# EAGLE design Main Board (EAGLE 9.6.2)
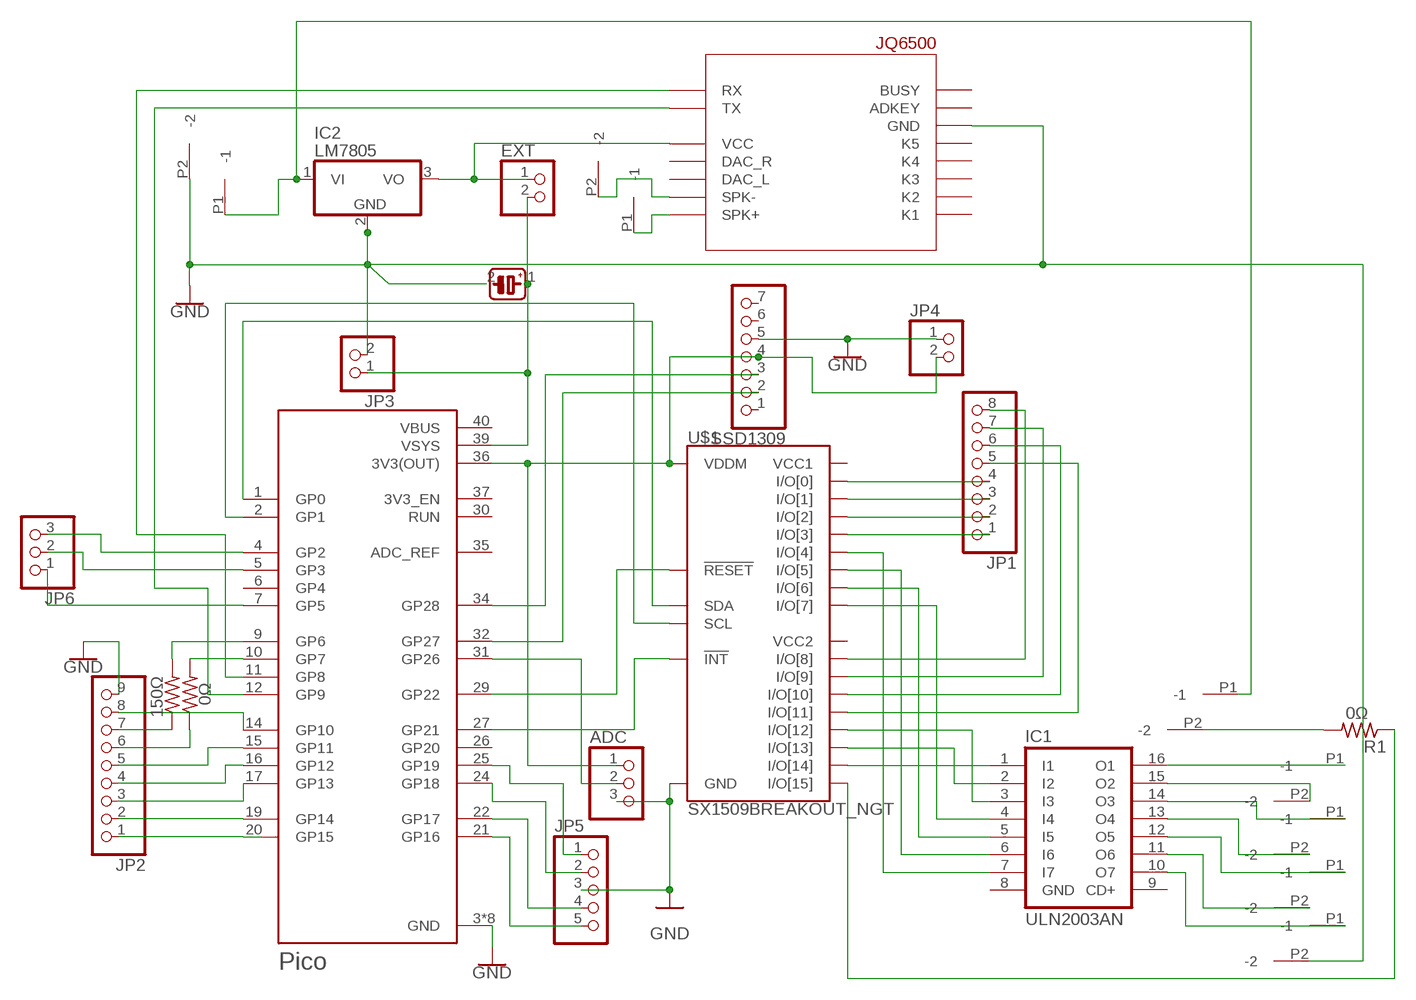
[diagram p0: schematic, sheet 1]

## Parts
ADC  PINHD-1X3  [1X03]
EXT  PINHD-1X2  [1X02]
IC1  ULN2003AN  [DIL16]
IC2  LM7805  7805TV  [TO220V]
JP1  PINHD-1X8  [1X08]
JP2  PINHD-1X9  [1X09]
JP3  PINHD-1X2  [1X02]
JP4  PINHD-1X2  [1X02]
JP5  PINHD-1X5  [1X05]
JP6  PINHD-1X3  [1X03]
R1  0Ω  R-US_0207/15  [0207/15]
R3  150Ω  R-US_0207/12  [0207/12]
R4  0Ω  R-US_0207/12  [0207/12]
SSD1309  PINHD-1X7  [1X07]
U1  Pico  RASPBERRY_PICOTH  [PICO-PKG-TH]
U$1  SX1509BREAKOUT_NGT  [BREAKOUT_NGT]
U$2  JQ6500  [JQ6500]
U$3  CONNECTORSCREWLESS2POS  [CONNECTORSCREWLESS2POS]
U$4  CONNECTORSCREWLESS2POS  [CONNECTORSCREWLESS2POS]
U$5  CONNECTORSCREWLESS2POS  [CONNECTORSCREWLESS2POS]
U$6  CONNECTORSCREWLESS2POS  [CONNECTORSCREWLESS2POS]
U$7  CONNECTORSCREWLESS2POS  [CONNECTORSCREWLESS2POS]
U$8  CONNECTORSCREWLESS2POS  [CONNECTORSCREWLESS2POS]
U$9  CONNECTORSCREWLESS2POS  [CONNECTORSCREWLESS2POS]
U$10  CAPACITOR_TANTALUM_RADIAL_10UF  [CAPACITOR_TANTALUM_RADIAL_10UF]

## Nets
GND: ADC.3 IC2.2(GND) JP2.9 JP3.2 JP4.1 JP5.3 SSD1309.5 U1.3(GND) U1.8(GND) U1.13(GND) U1.18(GND) U1.23(GND) U1.28(GND) U1.33(GND) U1.38(GND) U$1.GND U$1.GND3(GND) U$1.GND4(GND) U$2.GND1(GND) U$2.GND2(GND) U$3.P2(-2) U$8.P2(-2) U$10.2
N$1: JP1.4 U$1.I/O[0]
N$2: JP1.3 U$1.I/O[1]
N$3: JP1.1 U$1.I/O[3]
N$4: JP1.2 U$1.I/O[2]
N$5: JP1.8 U$1.I/O[8]
N$6: JP1.5 U$1.I/O[11]
N$7: JP1.7 U$1.I/O[9]
N$8: JP1.6 U$1.I/O[10]
N$9: IC1.3(I3) U$1.I/O[12]
N$10: IC1.2(I2) U$1.I/O[13]
N$11: IC1.1(I1) U$1.I/O[14]
N$12: IC1.4(I4) U$1.I/O[7]
N$13: IC1.5(I5) U$1.I/O[6]
N$14: IC1.6(I6) U$1.I/O[5]
N$15: IC1.7(I7) U$1.I/O[4]
N$16: IC2.1(VI) U$7.P1(-1) U$8.P1(-1)
N$17: R1.2 U$7.P2(-2)
N$18: EXT.1 IC2.3(VO) U$2.VCC
N$19: R4.2 U1.10(GP7)
N$20: SSD1309.3 U1.34(GP28)
N$21: R1.1 U$1.I/O[15]
N$22: IC1.16(O1) U$6.P1(-1)
N$23: IC1.15(O2) U$6.P2(-2)
N$24: IC1.14(O3) U$5.P1(-1)
N$25: IC1.13(O4) U$5.P2(-2)
N$26: IC1.12(O5) U$4.P1(-1)
N$27: IC1.11(O6) U$4.P2(-2)
N$28: IC1.10(O7) U$3.P1(-1)
N$29: ADC.1 JP4.2 SSD1309.4 U1.36(3V3(OUT)) U$1.VDDM
N$30: U1.1(GP0) U$1.SDA
N$31: U1.2(GP1) U$1.SCL
N$32: SSD1309.2 U1.32(GP27)
N$33: ADC.2 U1.31(GP26)
N$34: U1.29(GP22) U$1.!RESET
N$35: U1.27(GP21) U$1.!INT
N$36: U1.11(GP8) U$2.RX
N$37: U1.12(GP9) U$2.TX
N$38: U$2.SPK+ U$9.P1(-1)
N$39: U$2.SPK- U$9.P2(-2)
N$40: JP2.1 U1.20(GP15)
N$41: JP2.2 U1.19(GP14)
N$42: JP2.3 U1.17(GP13)
N$43: JP2.4 U1.16(GP12)
N$44: JP2.5 U1.15(GP11)
N$45: JP2.6 R4.1
N$46: R3.2 U1.9(GP6)
N$47: JP6.3 U1.4(GP2)
N$48: EXT.2 JP3.1 U1.39(VSYS) U$10.1
N$49: JP2.7 R3.1
N$50: JP6.2 U1.5(GP3)
N$51: JP2.8 U1.14(GP10)
N$52: JP5.1 U1.25(GP19)
N$53: JP5.2 U1.24(GP18)
N$54: JP5.4 U1.22(GP17)
N$55: JP5.5 U1.21(GP16)
N$56: JP6.1 U1.7(GP5)
Unconnected: IC1.9(CD+) SSD1309.1 SSD1309.6 SSD1309.7 U1.6(GP4) U1.26(GP20) U1.30(RUN) U1.35(ADC_REF) U1.37(3V3_EN) U$1.VCC1 U$1.VCC2 U$2.ADKEY U$2.BUSY U$2.DAC-L(DAC_L) U$2.DAC-R(DAC_R) U$2.K1 U$2.K2 U$2.K3 U$2.K4 U$2.K5

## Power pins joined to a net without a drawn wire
GND: IC1.8(GND)
VBUS: U1.40(VBUS)

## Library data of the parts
ADC JP6 = pinhead:PINHD-1X3: PIN HEADER
EXT JP3 JP4 = pinhead:PINHD-1X2: PIN HEADER
IC1 = uln-udn:ULN2003A: DRIVER ARRAY
IC2 = linear:78*: Positive VOLTAGE REGULATOR Source: http://cache.national.com/ds/LM/LM78L05.pdf http://www.fairchildsemi.com/ds/LM/LM7805.pdf
JP1 = pinhead:PINHD-1X8: PIN HEADER
JP2 = pinhead:PINHD-1X9: PIN HEADER
JP5 = pinhead:PINHD-1X5: PIN HEADER
R1 R3 R4 = rcl:R-US_: RESISTOR, American symbol; SPICEPREFIX: R
SSD1309 = pinhead:PINHD-1X7: PIN HEADER
U1 = RpiPico:RASPBERRY_PICO: Raspberry Pi Pico
U$1 = SX1509 Breakout:SX1509BREAKOUT_NGT
U$2 = JQ6500:JQ6500: JQ6500 MP3 Module
U$3-U$9 = Williams:CONNECTORSCREWLESS2POS
U$10 = Williams:CAPACITOR_TANTALUM_RADIAL_10UF

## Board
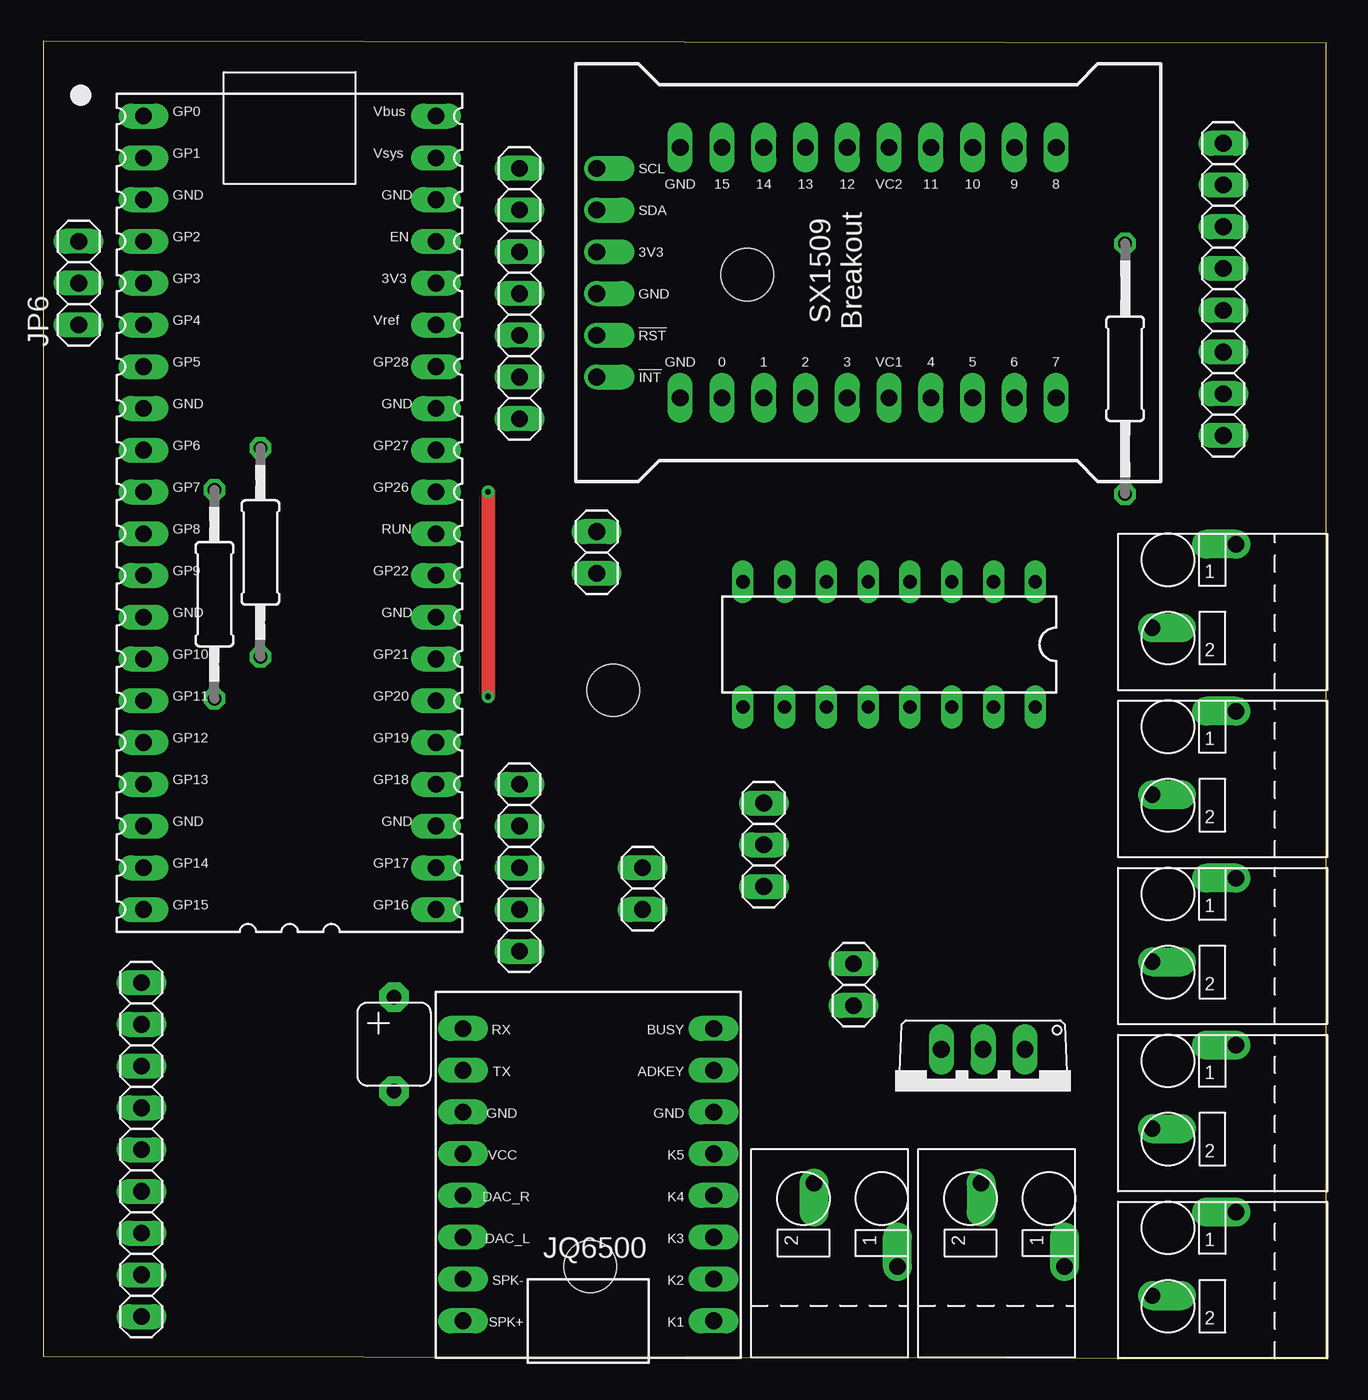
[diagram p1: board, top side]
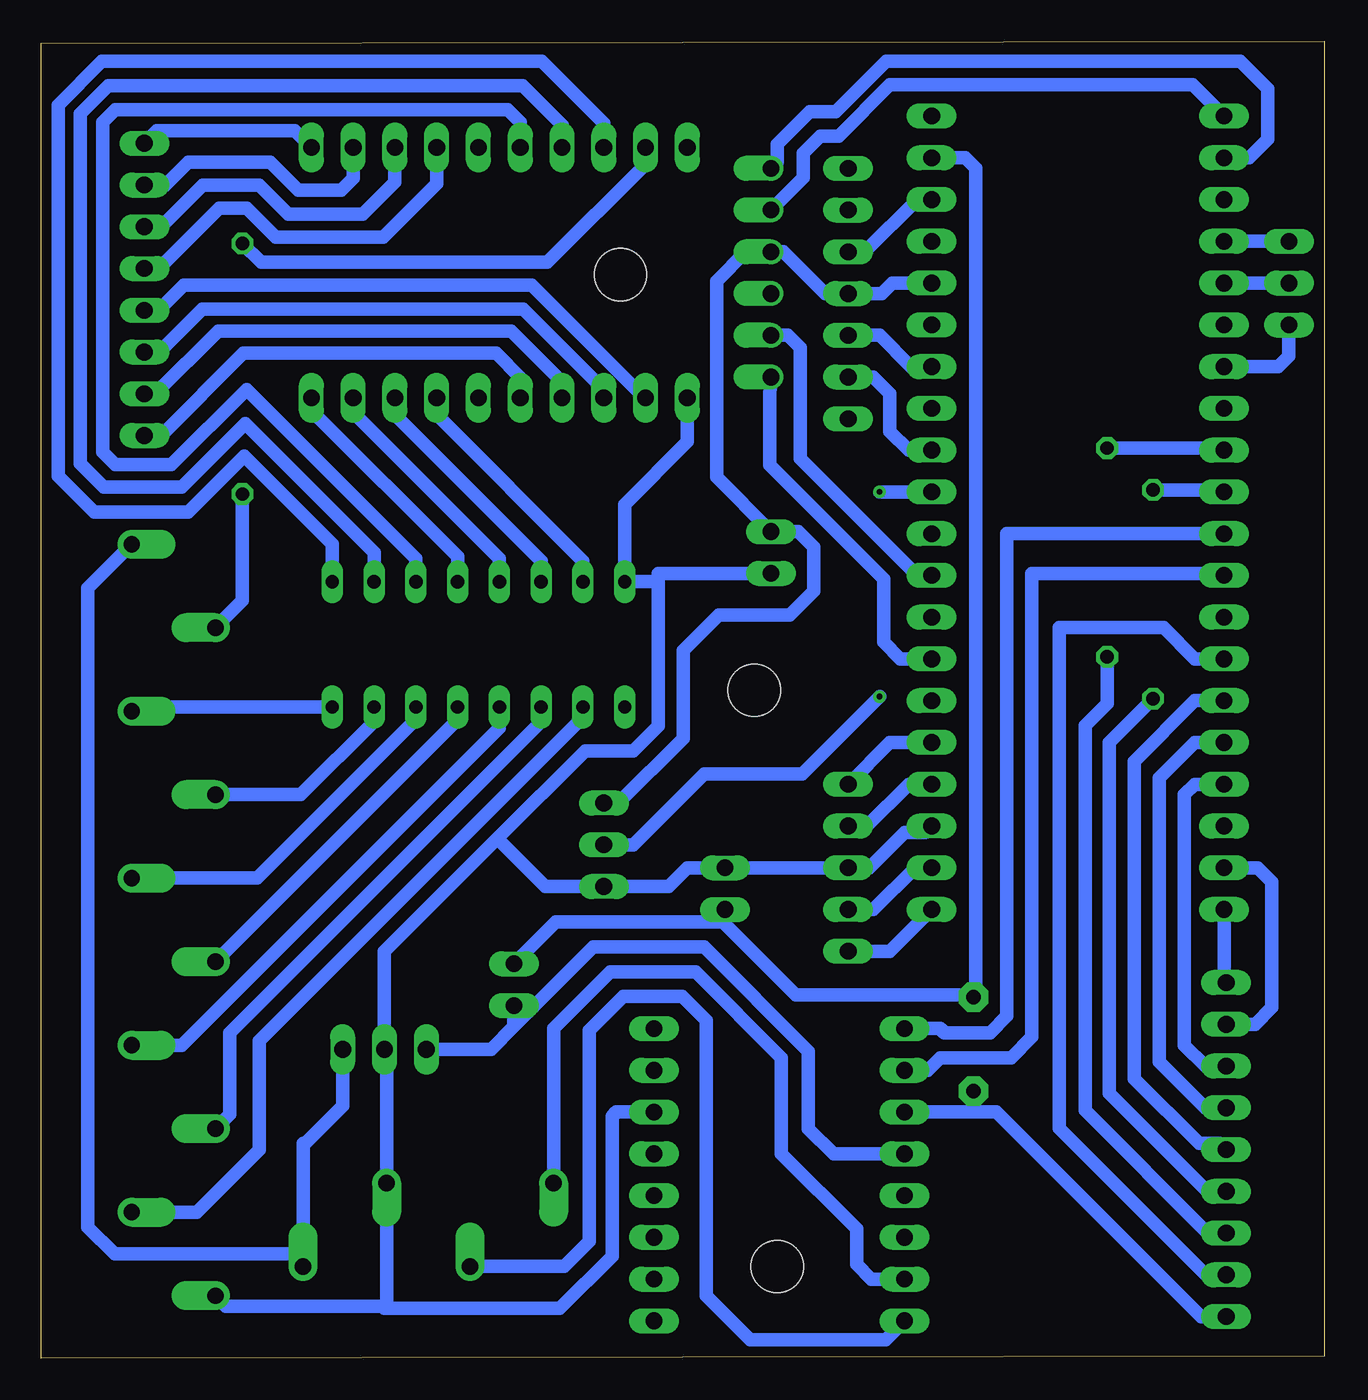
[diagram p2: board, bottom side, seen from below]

Size 78.03 x 80.13 mm. Coordinates in mm from the lower left corner, seen from the top.
Outline: 0,0.13 78.03,0 78.03,80 0,80.13 0,0.13
Copper layers (1*16): Top 0.035mm / dielectric 1.5mm / Bottom 0.035mm
Design rules "default *": minimum track width 6mil, minimum drill 0.35mm, track to track 6mil, track to pad 6mil, pad to pad 6mil, via to via 6mil, smd to smd 6mil, copper to edge 25mil, drill to drill 6mil, minimum pad ring 10mil, minimum via ring 8mil, stop-mask expansion 4mil, vias tented up to drill 0mil, thermal gap 10mil
Holes 3.17 mm at 34.67,40.64 42.8,65.91 33.27,5.59
tRestrict: area 29.9,35.9 to 39.4,45.4; area 38,61.2 to 47.6,70.7; area 28.5,0.8 to 38,10.4

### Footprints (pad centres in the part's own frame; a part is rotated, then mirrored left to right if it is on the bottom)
1X03 = drill 1.016 long: 1 -2.54,0; 2 0,0; 3 2.54,0
1X02 = drill 1.016 long: 1 -1.27,0; 2 1.27,0
DIL16 = drill 0.813 long: 1 -8.89,-3.81; 2 -6.35,-3.81; 3 -3.81,-3.81; 4 -1.27,-3.81; 5 1.27,-3.81; 6 3.81,-3.81; 7 6.35,-3.81; 8 8.89,-3.81; 9 8.89,3.81; 10 6.35,3.81; 11 3.81,3.81; 12 1.27,3.81; 13 -1.27,3.81; 14 -3.81,3.81; 15 -6.35,3.81; 16 -8.89,3.81
TO220V = drill 1.016 long: 1 -2.54,-2.54; 2 0,-2.54; 3 2.54,-2.54
1X08 = drill 1.016 long: 1 -8.89,0; 2 -6.35,0; 3 -3.81,0; 4 -1.27,0; 5 1.27,0; 6 3.81,0; 7 6.35,0; 8 8.89,0
1X09 = drill 1.016 long: 1 -10.16,0; 2 -7.62,0; 3 -5.08,0; 4 -2.54,0; 5 0,0; 6 2.54,0; 7 5.08,0; 8 7.62,0; 9 10.16,0
1X05 = drill 1.016 long: 1 -5.08,0; 2 -2.54,0; 3 0,0; 4 2.54,0; 5 5.08,0
0207/15 = drill 0.813 octagon: 1 -7.62,0; 2 7.62,0
0207/12 = drill 0.813 octagon: 1 -6.35,0; 2 6.35,0
1X07 = drill 1.016 long: 1 -7.62,0; 2 -5.08,0; 3 -2.54,0; 4 0,0; 5 2.54,0; 6 5.08,0; 7 7.62,0
PICO-PKG-TH = drill 1.016 long: 1 -8.89,24.13; 2 -8.89,21.59; 3 -8.89,19.05; 4 -8.89,16.51; 5 -8.89,13.97; 6 -8.89,11.43; 7 -8.89,8.89; 8 -8.89,6.35; 9 -8.89,3.81; 10 -8.89,1.27; 11 -8.89,-1.27; 12 -8.89,-3.81; 13 -8.89,-6.35; 14 -8.89,-8.89; 15 -8.89,-11.43; 16 -8.89,-13.97; 17 -8.89,-16.51; 18 -8.89,-19.05; 19 -8.89,-21.59; 20 -8.89,-24.13; 21 8.89,-24.13; 22 8.89,-21.59; 23 8.89,-19.05; 24 8.89,-16.51; 25 8.89,-13.97; 26 8.89,-11.43; 27 8.89,-8.89; 28 8.89,-6.35; 29 8.89,-3.81; 30 8.89,-1.27; 31 8.89,1.27; 32 8.89,3.81; 33 8.89,6.35; 34 8.89,8.89; 35 8.89,11.43; 36 8.89,13.97; 37 8.89,16.51; 38 8.89,19.05; 39 8.89,21.59; 40 8.89,24.13
BREAKOUT_NGT = drill 1.016 offset: !INT -6.35,15.24; !RESET -3.81,15.24; GND -1.27,15.24; SCL 6.35,15.24; SDA 3.81,15.24; VDDM 1.27,15.24 | drill 1.016 long: GND3 -7.62,10.16; GND4 7.62,10.16; I/O[0] -7.62,7.62; I/O[1] -7.62,5.08; I/O[2] -7.62,2.54; I/O[3] -7.62,0; I/O[4] -7.62,-5.08; I/O[5] -7.62,-7.62; I/O[6] -7.62,-10.16; I/O[7] -7.62,-12.7; I/O[8] 7.62,-12.7; I/O[9] 7.62,-10.16; I/O[10] 7.62,-7.62; I/O[11] 7.62,-5.08; I/O[12] 7.62,0; I/O[13] 7.62,2.54; I/O[14] 7.62,5.08; I/O[15] 7.62,7.62; VCC1 -7.62,-2.54; VCC2 7.62,-2.54
JQ6500 = drill 1.016 long: ADKEY -7.62,-6.35; BUSY -7.62,-8.89; DAC-L 7.62,3.81; DAC-R 7.62,1.27; GND1 -7.62,-3.81; GND2 7.62,-3.81; K1 -7.62,8.89; K2 -7.62,6.35; K3 -7.62,3.81; K4 -7.62,1.27; K5 -7.62,-1.27; RX 7.62,-8.89; SPK+ 7.62,8.89; SPK- 7.62,6.35; TX 7.62,-6.35; VCC 7.62,-1.27
CONNECTORSCREWLESS2POS = drill 1 pad 1.778 offset: P1 0,-5.08; P2 5.08,0
CAPACITOR_TANTALUM_RADIAL_10UF = drill 0.9 pad 1.778 octagon: 1 -2.54,0; 2 3.175,0

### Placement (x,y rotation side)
ADC  43.81,31.24 270 top
EXT  49.28,22.73 90 top
IC1  51.44,43.43 180 top
IC2  57.15,16.26 180 top
JP1  71.76,65.02 90 top
JP2  5.97,12.7 270 top
JP3  36.45,28.57 90 top
JP4  33.66,49.02 90 top
JP5  28.96,29.84 270 top
JP6  2.16,65.41 90 top
R1  65.79,60.2 270 top
R3  13.21,49.02 90 top
R4  10.41,46.48 90 top
SSD1309  28.96,64.77 90 top
U1  14.99,51.44 0 top
U$1  48.89,66.04 90 top
U$2  33.15,11.18 180 top
U$3  72.52,3.81 180 top
U$4  72.52,13.97 180 top
U$5  72.52,24.13 180 top
U$6  72.52,34.29 180 top
U$7  72.52,44.45 180 top
U$8  57.02,5.59 90 top
U$9  46.86,5.59 90 top
U$10  21.34,19.43 270 top

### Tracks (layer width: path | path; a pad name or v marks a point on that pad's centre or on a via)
GND
  Bottom 0.813: SSD1309.5 27.94,67.31 24.77,70.48 U1.38 | U$1.GND3 38.73,55.75 42.55,51.94 IC1.8 40.77,47.24 40.51,46.99 | 40.51,46.99 40.51,47.75 JP4.1 | 40.51,46.99 40.51,38.48 42.04,36.96 44.96,36.96 50.29,31.62 | 50.29,31.62 57.15,24.77 IC2.2 57.02,18.67 U$8.P2 57.02,3.17 | U$2.GND1 43.05,14.99 43.31,14.73 43.31,6.22 46.48,3.05 57.15,3.05 57.02,3.17 | U$2.GND2 21.21,14.99 | 21.21,14.99 19.94,14.99 7.49,2.54 JP2.9 | U1.23 24.26,32 25.53,32 27.69,29.84 JP5.3 JP3.2 38.73,29.84 39.88,28.7 ADC.3 47.37,28.7 50.29,31.62 | U$10.2 21.34,15.11 21.21,14.99 | 57.02,3.17 66.8,3.17 U$3.P2
N$1
  Bottom 0.813: U$1.I/O[0] 41.27,58.35 48.2,65.28 69.34,65.28 70.87,63.75 JP1.4
N$2
  Bottom 0.813: U$1.I/O[1] 43.81,58.93 48.72,63.83 68.22,63.83 70.83,61.21 JP1.3
N$3
  Bottom 0.813: U$1.I/O[3] 48.89,59.66 50.37,61.14 65.73,61.14 70.74,56.13 JP1.1 71.08,56.13
N$4
  Bottom 0.813: U$1.I/O[2] 46.35,59.4 49.44,62.48 67.26,62.48 71.07,58.67 JP1.2 71.63,58.55 71.12,58.55
N$5
  Bottom 0.813: JP1.8 70.99,74.68 62.61,74.68 U$1.I/O[8]
N$6
  Bottom 0.813: U$1.I/O[11] 53.98,71.44 57.22,68.2 63.75,68.2 65.53,69.98 67.18,69.98 70.87,66.29 JP1.5
N$7
  Bottom 0.813: U$1.I/O[9] 59.05,71.78 59.77,71.07 62.4,71.07 64.1,72.77 69.09,72.77 70.48,71.37 JP1.7
N$8
  Bottom 0.813: U$1.I/O[10] 56.52,71.54 58.46,69.6 62.99,69.6 64.77,71.37 68.2,71.37 70.74,68.83 JP1.6
N$9
  Bottom 0.813: U$1.I/O[12] 48.89,75.18 49.66,75.95 73.53,75.95 74.3,75.18 74.3,55.12 73.53,54.36 70.1,54.36 65.53,58.93 55.24,48.64 IC1.3
N$10
  Bottom 0.813: U$1.I/O[13] 46.35,75.03 48.75,77.42 73.93,77.42 75.64,75.71 75.64,54.43 74.22,53.01 69.47,53.01 65.62,56.86 57.78,49.02 IC1.2
N$11
  Bottom 0.813: U$1.I/O[14] 43.81,75.12 47.59,78.89 74.33,78.89 76.99,76.24 76.99,53.68 74.79,51.49 69.07,51.49 65.67,54.88 60.32,49.53 IC1.1
N$12
  Bottom 0.813: IC1.4 52.7,48.77 61.59,57.66 U$1.I/O[7]
N$13
  Bottom 0.813: U$1.I/O[6] 59.05,57.53 50.16,48.64 IC1.5
N$14
  Bottom 0.813: IC1.6 47.62,48.51 56.52,57.4 U$1.I/O[5]
N$15
  Bottom 0.813: IC1.7 45.09,48.51 53.98,57.4 U$1.I/O[4]
N$16
  Bottom 0.813: IC2.1 59.69,15.37 61.98,13.08 62.1,13.07 U$8.P1 62.61,6.35 73.55,6.35 75.18,7.99 75.18,46.86 U$7.P1
N$17
  Bottom 0.813: R1.2 65.79,46.1 U$7.P2
N$18
  Bottom 0.813: 49.28,20.19 50.67,18.8 IC2.3 | 49.28,20.19 44.45,25.02 37.72,25.02 31.37,18.67 31.37,13.97 29.84,12.45 U$2.VCC | EXT.1 49.28,20.19
N$19
  Bottom 0.813: R4.2 6.22,52.83 U1.10
N$20
  Bottom 0.813: U1.34 25.15,60.33 27.05,62.23 SSD1309.3
N$21
  Bottom 0.813: U$1.I/O[15] 41.27,72.64 47.24,66.67 64.64,66.67 R1.1
N$22
  Bottom 0.813: IC1.16 72.26,39.62 U$6.P1
N$23
  Bottom 0.813: IC1.15 57.78,38.73 62.23,34.29 U$6.P2
N$24
  Bottom 0.813: IC1.14 55.24,38.86 64.9,29.21 U$5.P1
N$25
  Bottom 0.813: IC1.13 52.7,38.86 U$5.P2
N$26
  Bottom 0.813: IC1.12 50.16,38.35 69.47,19.05 U$4.P1
N$27
  Bottom 0.813: U$4.P2 66.55,14.86 66.55,19.81 47.62,38.73 IC1.11
N$28
  Bottom 0.813: U$3.P1 68.58,8.89 64.77,12.7 64.77,19.3 45.34,38.73 45.34,39.37 IC1.10
N$29
  Bottom 0.813: U1.36 26.29,65.41 26.92,64.77 SSD1309.4 30.35,64.77 32.89,67.31 U$1.VDDM 35.18,67.31 36.96,65.53 36.96,53.59 JP4.2 32,50.29 31.05,49.34 31.05,46.67 32.51,45.21 36.83,45.21 38.99,43.05 38.99,37.72 42.93,33.78 ADC.1
N$30
  Bottom 0.813: U1.1 8,77.47 26.42,77.47 29.54,74.35 30.65,74.35 31.67,73.32 31.67,71.83 U$1.SDA
N$31
  Bottom 0.813: U1.2 4.57,73.03 3.43,74.17 3.43,77.22 5.12,78.91 26.63,78.91 29.72,75.82 31.3,75.82 33.27,73.84 33.27,72.77 U$1.SCL
N$32
  Bottom 0.813: U1.32 25.27,55.24 26.42,56.39 26.42,58.67 27.43,59.69 SSD1309.2
N$33  (via drill 0.35)
  Top 0.813: v27.05,52.7 v27.05,40.26
  Bottom 0.813: U1.31 v27.05,52.7 | v27.05,40.26 31.75,35.56 37.72,35.56 42.04,31.24 ADC.2
N$34
  Bottom 0.813: U1.29 24.77,47.62 31.88,54.74 31.88,59.69 31.88,60.07 31.88,61.47 32.64,62.23 U$1.!RESET
N$35
  Bottom 0.813: 24.73,42.55 U1.27 25.78,42.55 26.8,43.56 26.8,47.4 33.73,54.34 33.73,58.6 U$1.!INT
N$36
  Bottom 0.813: U1.11 19.3,50.16 19.3,20.83 20.32,19.81 23.11,19.81 23.37,20.07 U$2.RX
N$37
  Bottom 0.813: U1.12 6.22,47.75 17.78,47.75 17.78,19.56 19.05,18.29 23.37,18.29 24.13,17.53 U$2.TX
N$38
  Bottom 0.813: U$9.P1 46.23,5.59 44.7,7.11 44.7,19.94 42.62,22.02 39.04,22.02 37.59,20.57 37.59,3.81 34.92,1.14 26.67,1.14 U$2.SPK+
N$39
  Bottom 0.813: U$9.P2 46.86,20.07 43.43,23.5 38.23,23.5 33.02,18.29 33.02,12.45 28.45,7.87 28.45,5.71 27.56,4.83 U$2.SPK- 26.54,4.83
N$40
  Bottom 0.813: JP2.1 6.1,22.99 U1.20
N$41
  Bottom 0.813: U1.19 4.06,29.84 3.2,28.98 3.2,21.34 4.22,20.32 JP2.2
N$42
  Bottom 0.813: U1.17 7.87,34.92 8.51,34.29 8.51,19.05 7.24,17.78 JP2.3
N$43
  Bottom 0.813: U1.16 7.87,37.47 10.03,35.31 10.03,18.03 7.24,15.24 JP2.4
N$44
  Bottom 0.813: U1.15 7.87,40.01 11.56,36.32 11.56,17.02 7.62,13.08 6.35,13.08 JP2.5
N$45
  Bottom 0.813: JP2.6 7.11,10.16 13.08,16.13 13.08,37.47 R4.1
N$46
  Bottom 0.813: R3.2 6.22,55.37 U1.9
N$47
  Bottom 0.813: JP6.3 U1.4
N$48
  Bottom 0.813: U1.39 21.83,73.03 21.21,72.4 21.21,22.1 | EXT.2 46.74,26.54 36.58,26.54 | 36.58,26.54 35.62,25.59 32.13,22.1 21.21,22.1 | 36.58,26.54 36.89,26.86 JP3.1 | 21.21,22.1 U$10.1
N$49
  Bottom 0.813: JP2.7 7.08,7.62 14.55,15.09 14.55,24.13 | R3.1 13.21,39.85 14.55,38.5 14.55,24.13 | 14.55,24.13
N$50
  Bottom 0.813: JP6.2 U1.5
N$51
  Bottom 0.813: JP2.8 6.04,5.16 7.28,5.16 16.13,14.01 16.13,44.45 9.78,44.45 7.87,42.55 U1.14
N$52
  Bottom 0.813: U1.25 26.42,37.47 JP5.1
N$53
  Bottom 0.813: U1.24 25.27,34.92 27.81,32.38 JP5.2
N$54
  Bottom 0.813: U1.22 24.89,29.84 27.43,27.3 JP5.4
N$55
  Bottom 0.813: U1.21 26.42,24.77 JP5.5
N$56
  Bottom 0.813: JP6.1 2.16,60.96 2.79,60.33 U1.7

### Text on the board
Document: Keypad | 8 | CLK | 9 | 10 | Cols | GND | 11 | 3V3 | 0 | RST | 1 | MOSI | DC | CS | 2 | Rows | 3 | 3V3 | GND | 12V | TRI | Red | G1 | Wheel 3V3 | White | G2 | Wheel ADC | GND | GND | Wheel GND | Blue | G3 | 5V | G4 | HR | Rocker 1A | Ext 5V | Rocker 1B | Rocker 2A | HL | Rocker 2B | SPK | GND | 12V | - | + | SR | Green Ring Btn | Green Ring LED | Green Btn LED | SL | Black Btn | GND | GND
